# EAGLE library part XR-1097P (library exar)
EQUALIZER DISPLAY/FILTER/ADC
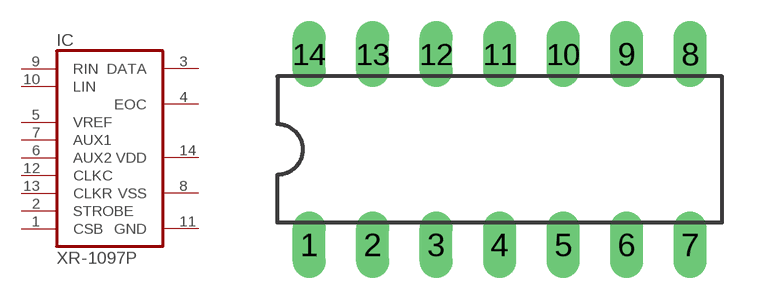
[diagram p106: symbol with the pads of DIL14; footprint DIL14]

Designator prefix IC

## XR-1097P (OC_FARNELL: unknown; OC_NEWARK: unknown)  [DIL14]
1  CSB  in
2  STROBE  in
3  DATA
4  EOC  out
5  VREF  in
6  AUX2  in
7  AUX1  in
8  VSS  pwr
9  RIN  in
10  LIN  in
11  GND  pwr
12  CLKC  in
13  CLKR  in
14  VDD  pwr

## Footprint DIL14 (pad centres in mm)
Dual In Line Package
drill 0.813 long: 1 -7.62,-3.81; 2 -5.08,-3.81; 3 -2.54,-3.81; 4 0,-3.81; 5 2.54,-3.81; 6 5.08,-3.81; 7 7.62,-3.81; 8 7.62,3.81; 9 5.08,3.81; 10 2.54,3.81; 11 0,3.81; 12 -2.54,3.81; 13 -5.08,3.81; 14 -7.62,3.81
